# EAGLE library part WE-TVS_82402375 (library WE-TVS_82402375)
TVS Diode Array WE-TVS, Standard Series - Low capazity - No leakage current - Low clamping voltage - high ESD voltage protection - Uni- and bidirectional protection -- DC Distribution -- Headsets and Accessoires -- PDAs -- Digital Cameras -- MP3-Players -- Touch Panels
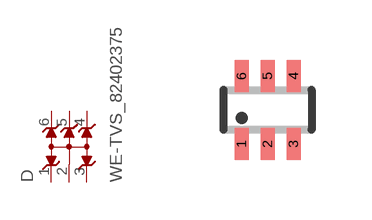
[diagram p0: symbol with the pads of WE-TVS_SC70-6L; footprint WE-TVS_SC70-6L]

Designator prefix D

## WE-TVS_82402375 (MPN: 82402375; OC_FARNELL: 1825868; OC_NEWARK: 79R6957; PACKAGE: SC70-6L; SUPPLIER: Wuerth Elektronik)  [WE-TVS_SC70-6L]
1  1  pas
2  GND  pwr
3  2  pas
4  3  pas
5  4  pas
6  5  pas

## Footprint WE-TVS_SC70-6L (pad centres in mm)
TVS Diode Array WE-TVS
smd 0.35 x 0.8: 1 -0.65,-0.85; 2 0,-0.85; 3 0.65,-0.85; 4 0.65,0.85; 5 0,0.85; 6 -0.65,0.85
